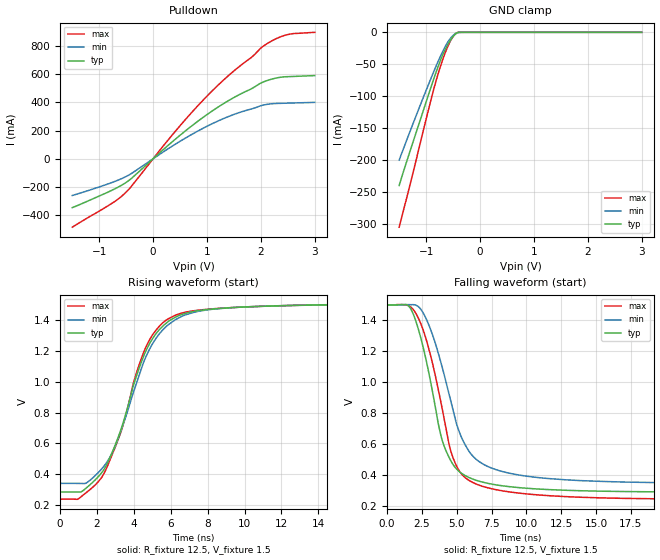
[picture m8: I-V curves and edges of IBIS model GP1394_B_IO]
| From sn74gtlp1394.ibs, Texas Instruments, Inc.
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[Model]   GP1394_B_IO
Model_type  I/O_open_drain
Vinh=   1.05
Vinl=   0.95
Vref =   1.5
Rref =   12.5
Cref =   30p
Vmeas =   1
| variable   typ   min   max
C_comp   7.23pF   5.84pF   8.17pF
| C_pulldown   8.33pF   5.92pF   11.32pF
| C_tri-state   7.23pF   5.84pF   8.17pF
[Temperature Range]   40   100   -40
| Ambient temperature   25   85   -40
[Voltage range]   3.3   3.15   3.45
[Pullup Reference]   1.5   1.5   1.5
[POWER Clamp Reference]   1.5   1.5   1.5
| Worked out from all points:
|   slope of the pulldown table from 0 to 0.225 V, typ, clamps not added: 2.91 ohm
|   GND clamp passes 1 mA (typ) near -0.42 V on its own axis
|   rising waveform, R_fixture 12.5, V_fixture 1.5: 20-80 % time 2.13ns typ, 2.17ns min, 2.05ns max; typ from 0.285 V to 1.5 V
|   falling waveform, R_fixture 12.5, V_fixture 1.5: 20-80 % time 1.86ns typ, 2.32ns min, 1.91ns max; typ from 1.5 V to 0.286 V
[GND Clamp]
| GP1394_B_IO
|   Voltage   I(typ)   I(min)   I(max)
-1.5V     -239.3mA   -199.7mA   -304.4mA
-1.26V    -175.9mA   -146.5mA   -225.3mA
-950mV    -96.07mA   -80.4mA    -118.9mA
-795mV    -57.7mA    -48.95mA   -69.94mA
-695mV    -35.82mA   -30.5mA    -43.5mA
-605mV    -20.14mA   -16.33mA   -23.65mA
-525mV    -9.339mA   -7.08mA    -10.04mA
-450mV    -2.421mA   -1.706mA   -1.925mA
-410mV    -478.4uA   -327.7uA   -148uA
-355mV    -24.86uA   -50.4uA    -20.08uA
3V        1.065nA    4.938nA    7.735nA
[Pulldown]
| GP1394_B_IO
|   Voltage   I(typ)   I(min)   I(max)
-1.5V     -346.7mA   -260.6mA   -485.2mA
-750mV    -220.8mA   -166.4mA   -312.7mA
-520mV    -172.7mA   -129.5mA   -243.8mA
-405mV    -140.3mA   -105.2mA   -196.4mA
375mV     126.8mA    94.55mA    177.9mA
860mV     274.8mA    202.9mA    388.5mA
1.4V      413mA      300mA      590.7mA
1.83V     498.1mA    354.2mA    721.2mA
2.01V     539.3mA    377.9mA    789.1mA
2.23V     568.3mA    391.4mA    842.1mA
2.455V    582.2mA    394.5mA    877.1mA
3V        590.5mA    400.3mA    897.5mA
[Ramp]
| GP1394_B_IO
| variable   typ   min   max
dV/dt_r   0.73/2.13E-09   0.70/2.20E-09   0.76/2.07E-09
dV/dt_f   0.73/1.86E-09   0.70/2.33E-09   0.76/1.93E-09
R_load = 12.5
[Rising Waveform]
| GP1394_B_IO
R_fixture =   12.5
C_fixture =   0
L_fixture =   0
V_fixture =   1.5
V_fixture_min = 1.5
V_fixture_max = 1.5
|   Time   V(typ)   V(min)   V(max)
0s        284.8mV    340.8mV    238.6mV
1.16ns    287.3mV    340.3mV    256.9mV
2.465ns   449.8mV    466.7mV    426.5mV
3.32ns    698.2mV    690mV      682.6mV
3.985ns   980.8mV    934.8mV    996.2mV
4.635ns   1.196V     1.157V     1.22V
5.385ns   1.338V     1.311V     1.36V
6.24ns    1.417V     1.401V     1.43V
10.29ns   1.485V     1.486V     1.486V
24.99ns   1.5V       1.5V       1.5V
[Falling Waveform]
| GP1394_B_IO
R_fixture =   12.5
C_fixture =   0
L_fixture =   0
V_fixture =   1.5
V_fixture_min = 1.5
V_fixture_max = 1.5
|   Time   V(typ)   V(min)   V(max)
0s        1.5V       1.5V       1.5V
1.59ns    1.489V     1.502V     1.493V
2.605ns   1.221V     1.447V     1.335V
3.29ns    924.9mV    1.3V       1.111V
4.07ns    592.7mV    1.059V     776.1mV
4.835ns   453.4mV    784.2mV    487.5mV
5.945ns   379.2mV    543.3mV    359.8mV
7.475ns   339.6mV    444mV      309.5mV
10.52ns   309mV      384.6mV    271.2mV
24.99ns   286.2mV    343.7mV    240.4mV
